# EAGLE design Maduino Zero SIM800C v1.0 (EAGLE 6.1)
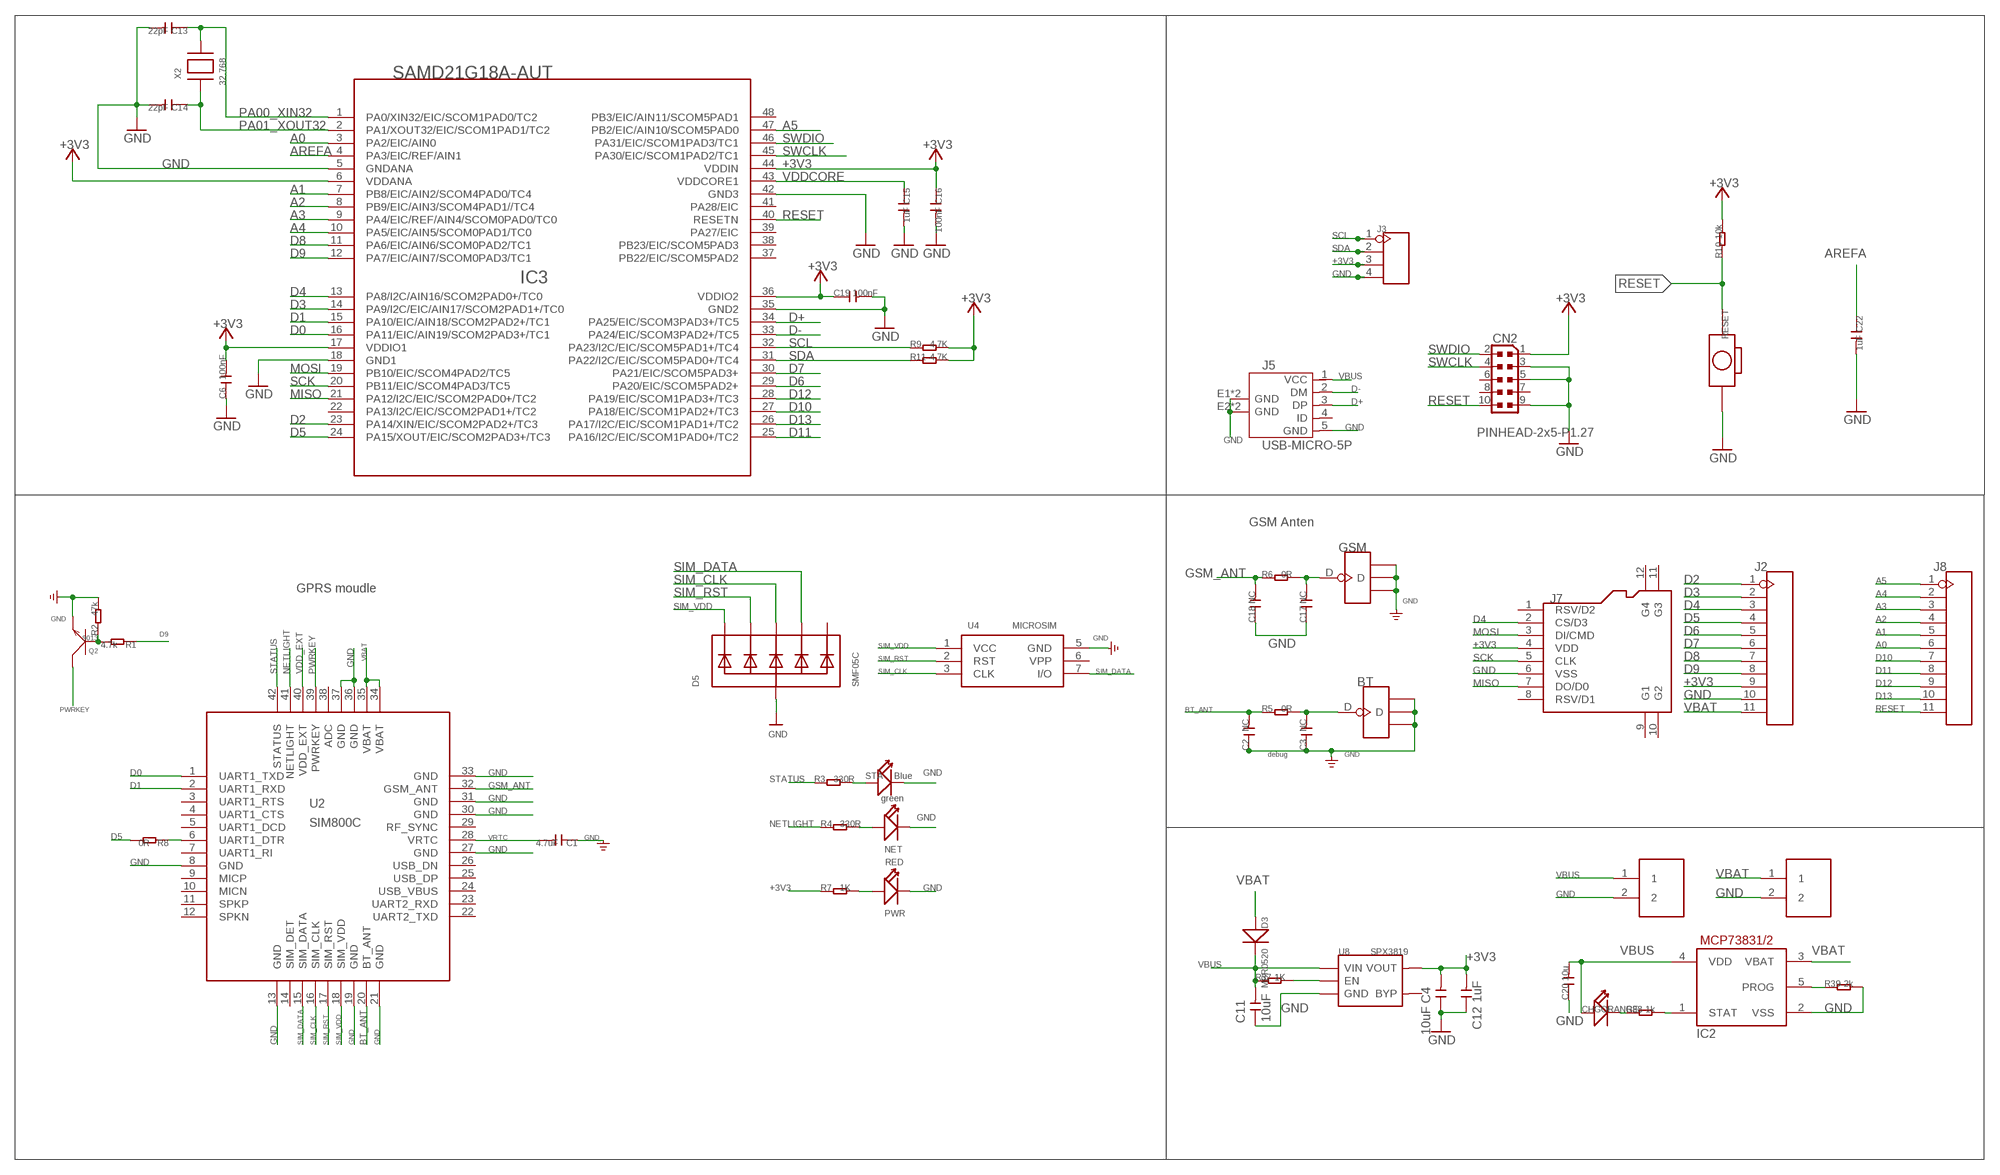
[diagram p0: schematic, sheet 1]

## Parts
BT  ANTENNA-U-FL  [4P-U-FL]
C1  4.7uF  C-0805  [C0805]
C2  NC  C-0402  [C0402]
C3  NC  C-0402  [C0402]
C4  10uF  C-0603  [C0603]
C6  100nF  C-0603  [C0603]
C11  10uF  C-0603  [C0603]
C12  1uF  C-0603  [C0603]
C13  22pF  C-0603  [C0603]
C14  22pF  C-0603  [C0603]
C15  1uF  C-0603  [C0603]
C16  100nF  C-0603  [C0603]
C17  NC  C-0402  [C0402]
C18  NC  C-0402  [C0402]
C19  100nF  C-0603  [C0603]
C20  10u  C-0603  [C0603]
C22  1uF  C-0603  [C0603]
CHG  ORANGE  007-LED0603  [D0603]
CN2  PINHEAD-2x5-P1.27  0171_PH127-205DF055G00AROUND-PADS  [PINHEAD_2X05_127]
D3  MBR0520  D'1206'  [SOD123]
D5  SMF05C  TVSARRAY_5LANE  [SOT363]
GSM  ANTENNA-U-FL  [4P-U-FL]
IC2  MCP73831/OT  [SOT23-5L]
IC3  SAMD21G18A-AUT  ATSAMD21G18A-AUT  [TQFP48-7X7]
J1  PH2.0-2P-90-DIP  [PH2.0-2P-90-DIP]
J2  HEADER-11P-2.54  [11P-2.54]
J3  HEADER-4P-60/35MILROUND  [4P-65/35ROUND]
J5  USB-MICRO-5P  [MICRO-USB-5P]
J6  PH2.0-2P-90-DIP  [PH2.0-2P-90-DIP]
J7  HOLDER-MICROSD-8P  [8P-SMD]
J8  HEADER-11P-2.54  [11P-2.54]
NET  green  LED'0603'  [LED-0603]
PWR  RED  LED'0603'  [LED-0603]
Q2  9013  TRANSISTOR-NPN-SOT23  [SOT23]
R1  4.7k  R-0603  [R0603]
R2  47k  R-0603  [R0603]
R3  330R  R-0603  [R0603]
R4  330R  R-0603  [R0603]
R5  0R  R-0603  [R0603]
R6  0R  R-0603  [R0603]
R7  1K  R-0603  [R0603]
R8  0R  R-0603  [R0603]
R9  4.7K  R-0603  [R0603]
R10  10k  R-0603  [R0603]
R11  4.7K  R-0603  [R0603]
R37  1K  R-0603  [R0603]
R38  1k  R-0603  [R0603]
R39  2k  R-0603  [R0603]
RESET  BOTTON-2P-90D  [2P-7.62X3.56-90D]
STA  Blue  LED'0603'  [LED-0603]
U2  SIM800C  [SIM800C]
U4  MICROSIM  [MICROSIM]
U8  SPX3819  [SOT23-5]
X2  32.768  XTAL-3.2X1.5  [XTAL3215]

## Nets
+3V3: C4.2 C6.2 C12.2 C16.1 C19.1 CN2.1 IC3.6(VDDANA) IC3.17(VDDIO1) IC3.36(VDDIO2) IC3.44(VDDIN) J2.9 J3.3 J7.4(VDD) R7.1 R9.2 R10.2 R11.2 U8.5(VOUT)
A0: IC3.3(PA2/EIC/AIN0) J8.6
A1: IC3.7(PB8/EIC/AIN2/SCOM4PAD0/TC4) J8.5
A2: IC3.8(PB9/EIC/AIN3/SCOM4PAD1//TC4) J8.4
A3: IC3.9(PA4/EIC/REF/AIN4/SCOM0PAD0/TC0) J8.3
A4: IC3.10(PA5/EIC/AIN5/SCOM0PAD1/TC0) J8.2
A5: IC3.47(PB2/EIC/AIN10/SCOM5PAD0) J8.1
AREFA: C22.1 IC3.4(PA3/EIC/REF/AIN1)
BT_ANT: C2.2 R5.1 U2.20(BT_ANT)
D0: IC3.16(PA11/EIC/AIN19/SCOM2PAD3+/TC1) U2.1(UART1_TXD)
D1: IC3.15(PA10/EIC/AIN18/SCOM2PAD2+/TC1) U2.2(UART1_RXD)
D2: IC3.23(PA14/XIN/EIC/SCOM2PAD2+/TC3) J2.1
D3: IC3.14(PA9/I2C/EIC/AIN17/SCOM2PAD1+/TC0) J2.2
D4: IC3.13(PA8/I2C/AIN16/SCOM2PAD0+/TC0) J2.3 J7.2(CS/D3)
D5: IC3.24(PA15/XOUT/EIC/SCOM2PAD3+/TC3) J2.4 R8.2
D6: IC3.29(PA20/EIC/SCOM5PAD2+) J2.5
D7: IC3.30(PA21/EIC/SCOM5PAD3+) J2.6
D8: IC3.11(PA6/EIC/AIN6/SCOM0PAD2/TC1) J2.7
D9: IC3.12(PA7/EIC/AIN7/SCOM0PAD3/TC1) J2.8 R1.1
D10: IC3.27(PA18/EIC/SCOM1PAD2+/TC3) J8.7
D11: IC3.25(PA16/I2C/EIC/SCOM1PAD0+/TC2) J8.8
D12: IC3.28(PA19/EIC/SCOM1PAD3+/TC3) J8.9
D13: IC3.26(PA17/I2C/EIC/SCOM1PAD1+/TC2) J8.10
D+: IC3.34(PA25/EIC/SCOM3PAD3+/TC5) J5.3(DP)
D-: IC3.33(PA24/EIC/SCOM3PAD2+/TC5) J5.2(DM)
GND: BT.GND1 BT.GND2 BT.GND3 C1.1 C2.1 C3.1 C4.1 C6.1 C11.1 C12.1 C13.2 C14.2 C15.2 C16.2 C17.1 C18.1 C19.2 C20.1 C22.2 CN2.3 CN2.5 CN2.9 D5.2(A) GSM.GND1 GSM.GND2 GSM.GND3 IC2.2(VSS) IC3.5(GNDANA) IC3.18(GND1) IC3.35(GND2) IC3.42(GND3) J1.2 J2.10 J3.4 J5.5(GND) J5.E1(GND) J5.E2(GND) J5.P1(GND) J5.P2(GND) J6.2 J7.6(VSS) NET.- PWR.- Q2.2(E) R2.2 R39.2 RESET.P$2 STA.- U2.8(GND) U2.13(GND) U2.19(GND) U2.21(GND) U2.27(GND) U2.30(GND) U2.31(GND) U2.33(GND) U2.36(GND) U2.37(GND) U4.5(GND) U8.2(GND)
GSM_ANT: C18.2 R6.1 U2.32(GSM_ANT)
MISO: IC3.21(PA12/I2C/EIC/SCOM2PAD0+/TC2) J7.7(DO/D0)
MOSI: IC3.19(PB10/EIC/SCOM4PAD2/TC5) J7.3(DI/CMD)
N$1: NET.+ R4.2
N$2: R8.1 U2.6(UART1_DTR)
N$3: PWR.+ R7.2
N$7: R3.2 STA.+
N$24: R37.2 U8.3(EN)
N$25: CHG.- R38.1
N$26: IC2.1(STAT) R38.2
N$28: BT.D C3.2 R5.2
N$31: IC2.5(PROG) R39.1
N$36: Q2.1(B) R1.2 R2.1
N$94: C17.2 GSM.D R6.2
NETLIGHT: R4.1 U2.41(NETLIGHT)
PA00_XIN32: C13.1 IC3.1(PA0/XIN32/EIC/SCOM1PAD0/TC2) X2.P$2
PA01_XOUT32: C14.1 IC3.2(PA1/XOUT32/EIC/SCOM1PAD1/TC2) X2.P$1
PWRKEY: Q2.3(C) U2.39(PWRKEY)
RESET: CN2.10 IC3.40(RESETN) J8.11 R10.1 RESET.P$1
SCK: IC3.20(PB11/EIC/SCOM4PAD3/TC5) J7.5(CLK)
SCL: IC3.32(PA23/I2C/EIC/SCOM5PAD1+/TC4) J3.1 R9.1
SDA: IC3.31(PA22/I2C/EIC/SCOM5PAD0+/TC4) J3.2 R11.1
SIM_CLK: D5.4(C3) U2.16(SIM_CLK) U4.3(CLK)
SIM_DATA: D5.5(C4) U2.15(SIM_DATA) U4.7(I/O)
SIM_RST: D5.3(C2) U2.17(SIM_RST) U4.2(RST)
SIM_VDD: D5.1(C1) U2.18(SIM_VDD) U4.1(VCC)
STATUS: R3.1 U2.42(STATUS)
SWCLK: CN2.4 IC3.45(PA30/EIC/SCOM1PAD2/TC1)
SWDIO: CN2.2 IC3.46(PA31/EIC/SCOM1PAD3/TC1)
VBAT: D3.+ IC2.3(VBAT) J2.11 J6.1 U2.34(VBAT) U2.35(VBAT)
VBUS: C11.2 C20.2 CHG.+ D3.- IC2.4(VDD) J1.1 J5.1(VCC) R37.1 U8.1(VIN)
VDD_EXT: U2.40(VDD_EXT)
VDDCORE: C15.1 IC3.43(VDDCORE1)
VRTC: C1.2 U2.28(VRTC)
Unconnected: CN2.6 CN2.7 CN2.8 D5.6(C5) IC3.22(PA13/I2C/EIC/SCOM2PAD1+/TC2) IC3.37(PB22/EIC/SCOM5PAD2) IC3.38(PB23/EIC/SCOM5PAD3) IC3.39(PA27/EIC) IC3.41(PA28/EIC) IC3.48(PB3/EIC/AIN11/SCOM5PAD1) J5.4(ID) J7.1(RSV/D2) J7.8(RSV/D1) J7.9(G1) J7.10(G2) J7.11(G3) J7.12(G4) U2.3(UART1_RTS) U2.4(UART1_CTS) U2.5(UART1_DCD) U2.7(UART1_RI) U2.9(MICP) U2.10(MICN) U2.11(SPKP) U2.12(SPKN) U2.14(SIM_DET) U2.22(UART2_TXD) U2.23(UART2_RXD) U2.24(USB_VBUS) U2.25(USB_DP) U2.26(USB_DN) U2.29(RF_SYNC) U2.38(ADC) U4.6(VPP) U8.4(BYP)

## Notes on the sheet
- GSM Anten
- GPRS moudle
- debug

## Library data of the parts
BT GSM = Connector:ANTENNA-U-FL
C1-C4 C6 C11-C20 C22 = Discrete:C*: Ceramic Capacitors
CHG = Discrete:007-LED*
CN2 = Connettori:0171_PH127-205DF055G00A: 2x5 PASSO 1,27
D3 = Discrete:D*
D5 = microbuilder:TVSARRAY_5LANE: Voltage Transient Suppressor Array SOT363 SMF05C - 100W 5V: Digikey - SMF05CT1GOSCT-ND
IC2 = adafruit:MCP73831: MCP73831/2 Miniature Single-Cell, Fully Integrated Li-Ion, Li-Polymer Charge Management Controllers. Nice and small simple lipoly charge controller, with adjustable current and status output (LED) http://www.ladyada.net/library/pcb/eaglelibrary.html
IC3 = IC:ATSAMD21G18A-AUT: Atmel D21 32bit ARM Cortex-M0 microcontroller - 48 PIN TQFP 256KB flash memory + 32KB SRAM
J1 J6 = Connector:PH2.0-2P-90-DIP
J2 J8 = Connector:HEADER-11P
J3 = Connector:HEADER-4P
J5 = Connector:USB-MICRO-5P
J7 = Connector:HOLDER-MICROSD-8P
NET PWR STA = Discrete:LED*
Q2 = Discrete:TRANSISTOR-NPN*: NPN audion
R1-R11 R37-R39 = Discrete:R*
RESET = Discrete:BOTTON-2P
U2 = moudle:SIM800C
U4 = Connector:MICROSIM
U8 = IC:SPX3819
X2 = adafruit2:XTAL: Low cost SMT crystals, no capacitors included

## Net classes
0 default: width 0.152 mm, drill 0.152 mm, clearance 0.152 mm
2 gnd: width 0.305 mm, drill 0.559 mm, clearance 0.254 mm
3 usbvcc: width 0.508 mm, drill 0.61 mm, clearance 0.254 mm
4 USBpair: width 0.254 mm, drill 0.406 mm, clearance 0.406 mm

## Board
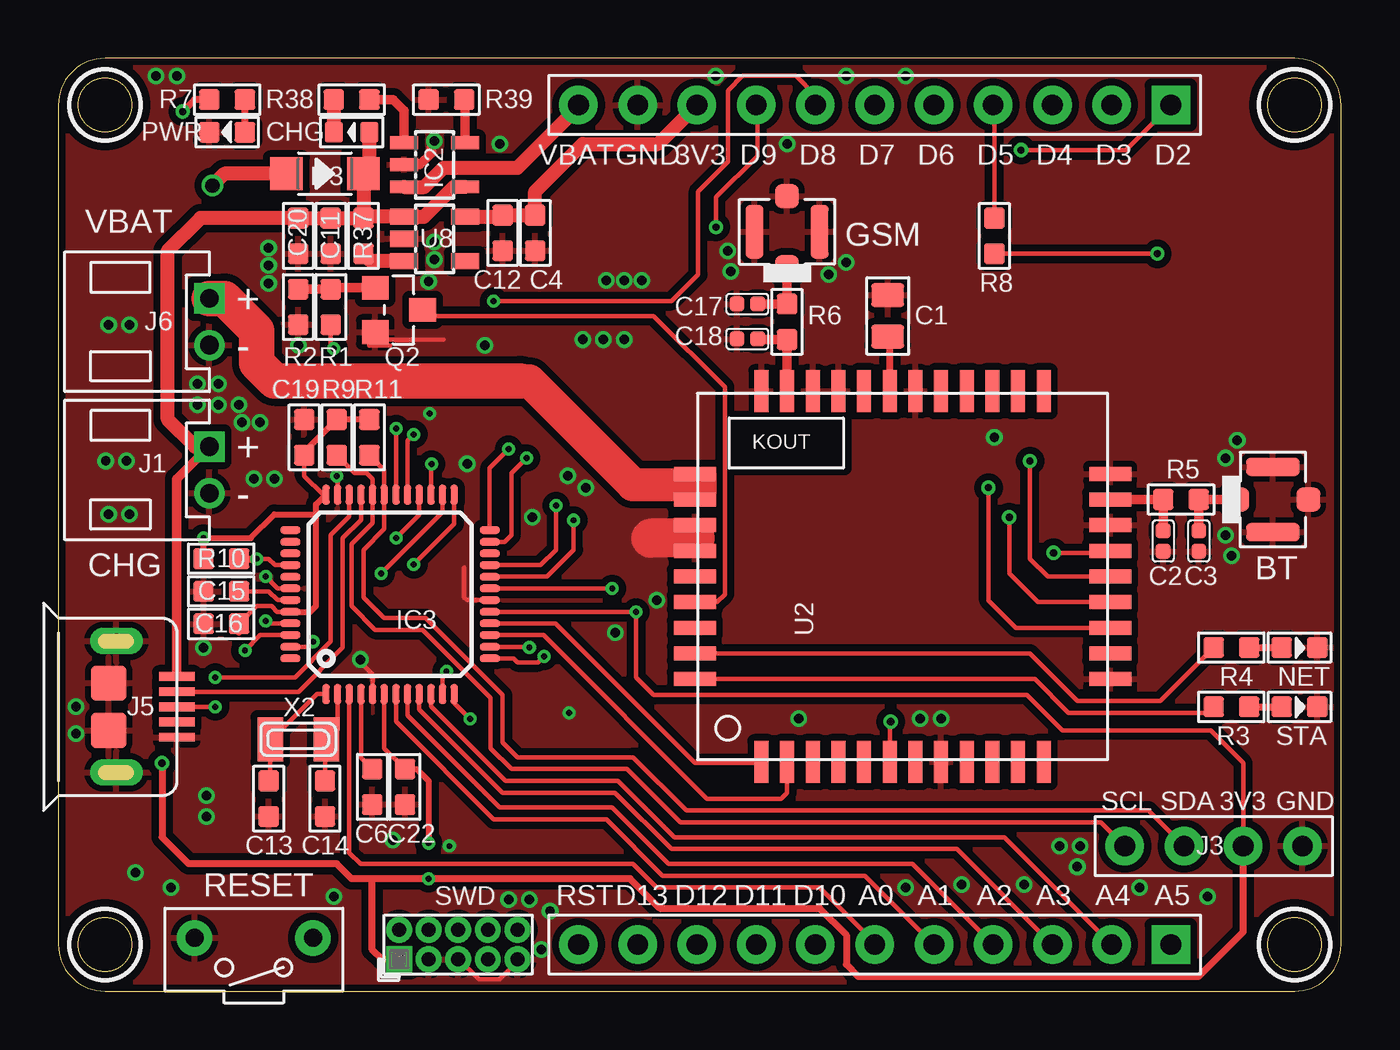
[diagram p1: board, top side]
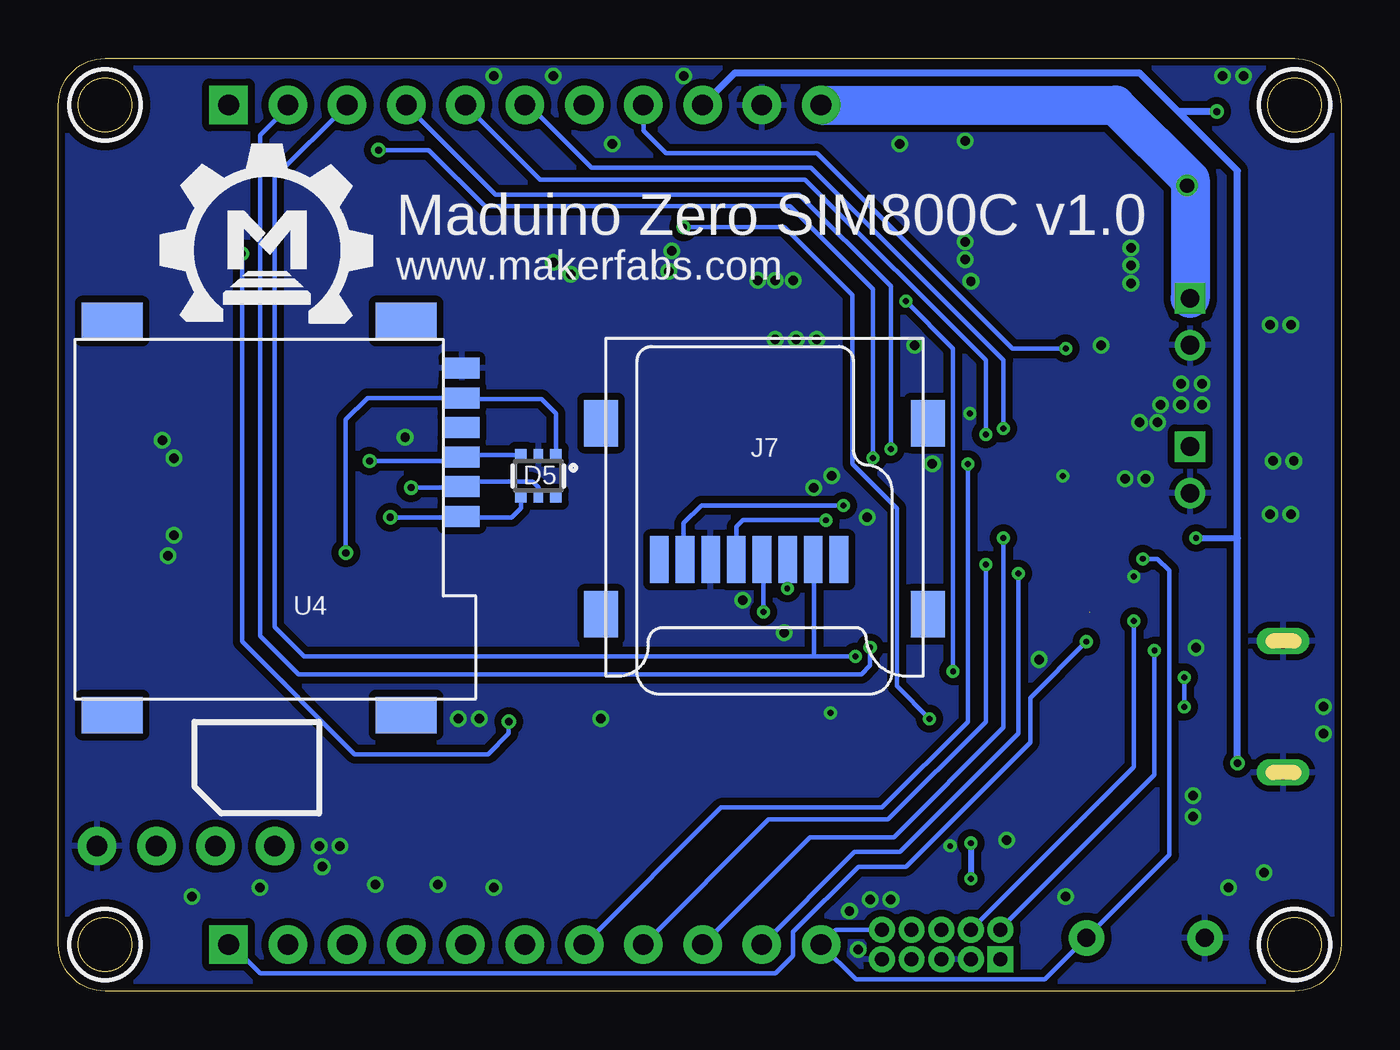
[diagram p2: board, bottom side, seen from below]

Size 55 x 40 mm. Coordinates in mm from the lower left corner, seen from the top.
Outline: 0,38 0,2 arc90 2,0 53,0 arc90 55,2 55,38 arc90 53,40 2,40 arc90 0,38
Outline: circle at 53,2 radius 1.14
Outline: circle at 53,38 radius 1.14
Outline: circle at 2,2 radius 1.14
Outline: circle at 2,38 radius 1.14
Copper layers (1*16): Top 0.035mm / dielectric 1.5mm / Bottom 0.035mm
Design rules: minimum track width 6mil, minimum drill 10mil, track to track 6mil, track to pad 6mil, pad to pad 6mil, via to via 6mil, smd to smd 0mil, copper to edge 10mil, drill to drill 10mil, minimum pad ring 10mil, minimum via ring 6mil, stop-mask expansion 2mil, vias tented up to drill 100mil, thermal gap 10mil
tRestrict: area 51.5,0.5 to 54.5,3.5; area 51.5,36.5 to 54.5,39.5; area 0.5,0.5 to 3.5,3.5; area 0.5,36.5 to 3.5,39.5
bRestrict: area 51.5,0.5 to 54.5,3.5; area 51.5,36.5 to 54.5,39.5; area 0.5,0.5 to 3.5,3.5; area 0.5,36.5 to 3.5,39.5

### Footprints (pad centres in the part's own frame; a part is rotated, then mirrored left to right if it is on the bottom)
4P-U-FL = smd 1.016 x 1.016: D -1.524,0; GND3 1.524,0 | smd 2.286 x 0.762: GND1 0,1.397; GND2 0,-1.397
C0805 = smd 1.016 x 1.397: 1 -0.889,0; 2 0.889,0
C0402 = smd 0.635 x 0.635: 1 -0.445,0; 2 0.445,0
C0603 = smd 0.889 x 0.889: 1 -0.762,0; 2 0.762,0
D0603 = smd 0.762 x 0.889: + -0.762,0; - 0.762,0
PINHEAD_2X05_127 = drill 0.6 pad 1.016 square: 1 -0.635,2.54 | drill 0.6 pad 1.016: 2 0.635,2.54; 3 -0.635,1.27; 4 0.635,1.27; 5 -0.635,0; 6 0.635,0; 7 -0.635,-1.27; 8 0.635,-1.27; 9 -0.635,-2.54; 10 0.635,-2.54
SOD123 = smd 1.397 x 1.397: + -1.651,0; - 1.651,0
SOT363 = smd 0.5 x 0.5: 1 -0.75,-0.9; 3 0.75,-0.9; 4 0.75,0.9; 6 -0.75,0.9 | smd 0.4 x 0.5: 2 0,-0.9; 5 0,0.9
SOT23-5L = smd 0.55 x 1.2: 1 -0.95,-1.3; 2 0,-1.3; 3 0.95,-1.3; 4 0.95,1.3; 5 -0.95,1.3
TQFP48-7X7 = smd 0.85 x 0.32: 1 -4.275,2.75; 2 -4.275,2.25; 3 -4.275,1.75; 4 -4.275,1.25; 5 -4.275,0.75; 6 -4.275,0.25; 7 -4.275,-0.25; 8 -4.275,-0.75; 9 -4.275,-1.25; 10 -4.275,-1.75; 11 -4.275,-2.25; 12 -4.275,-2.75; 25 4.275,-2.75; 26 4.275,-2.25; 27 4.275,-1.75; 28 4.275,-1.25; 29 4.275,-0.75; 30 4.275,-0.25; 31 4.275,0.25; 32 4.275,0.75; 33 4.275,1.25; 34 4.275,1.75; 35 4.275,2.25; 36 4.275,2.75 | smd 0.32 x 0.85: 13 -2.75,-4.275; 14 -2.25,-4.275; 15 -1.75,-4.275; 16 -1.25,-4.275; 17 -0.75,-4.275; 18 -0.25,-4.275; 19 0.25,-4.275; 20 0.75,-4.275; 21 1.25,-4.275; 22 1.75,-4.275; 23 2.25,-4.275; 24 2.75,-4.275; 37 2.75,4.275; 38 2.25,4.275; 39 1.75,4.275; 40 1.25,4.275; 41 0.75,4.275; 42 0.25,4.275; 43 -0.25,4.275; 44 -0.75,4.275; 45 -1.25,4.275; 46 -1.75,4.275; 47 -2.25,4.275; 48 -2.75,4.275
PH2.0-2P-90-DIP = drill 0.8 square: 1 0,1 | drill 0.8: 2 0,-1
11P-2.54 = drill 0.889 pad 1.651 square: 1 0,12.7 | drill 0.889 pad 1.651: 2 0,10.16; 3 0,7.62; 4 0,5.08; 5 0,2.54; 6 0,0; 7 0,-2.54; 8 0,-5.08; 9 0,-7.62; 10 0,-10.16; 11 0,-12.7
4P-65/35ROUND = drill 0.889 pad 1.651: 1 0,3.81; 2 0,1.27; 3 0,-1.27; 4 0,-3.81
MICRO-USB-5P = smd 0.38 x 1.52: 1 -1.3,0; 2 -0.65,0; 3 0,0; 4 0.65,0; 5 1.3,0 | smd 1.524 x 1.524: E1 -1.016,-2.921; E2 1.016,-2.921 | drill 0.635 pad 1.143 long: P1 -2.819,-2.591; P2 2.819,-2.591
8P-SMD = smd 0.8 x 2.008: 1 -3.198,0.254; 2 -2.098,0.254; 3 -0.998,0.254; 4 0.102,0.254; 5 1.202,0.254; 6 2.302,0.254; 7 3.402,0.254; 8 4.502,0.254 | smd 1.45 x 2: 9 -7.002,2.6; 10 7.002,2.6; 11 -7.002,-5.598; 12 7.002,-5.598
LED-0603 = smd 0.889 x 0.889: + -0.762,0; - 0.762,0
SOT23 = smd 1.016 x 1.143: 1 -0.95,-1.016; 2 0.95,-1.016; 3 0,1.016
R0603 = smd 0.889 x 0.889: 1 -0.762,0; 2 0.762,0
2P-7.62X3.56-90D = drill 0.762 pad 1.524: P$1 0,2.54; P$2 0,-2.54
SIM800C = smd 1.8 x 0.6: 1 -7.95,6.05; 2 -7.95,4.95; 3 -7.95,3.85; 4 -7.95,2.75; 5 -7.95,1.65; 6 -7.95,0.55; 7 -7.95,-0.55; 8 -7.95,-1.65; 9 -7.95,-2.75; 10 -7.95,-3.85; 11 -7.95,-4.95; 12 -7.95,-6.05; 22 7.95,-6.05; 23 7.95,-4.95; 24 7.95,-3.85; 25 7.95,-2.75; 26 7.95,-1.65; 27 7.95,-0.55; 28 7.95,0.55; 29 7.95,1.65; 30 7.95,2.75; 31 7.95,3.85; 32 7.95,4.95; 33 7.95,6.05 | smd 0.6 x 1.8: 13 -4.4,-8.9; 14 -3.3,-8.9; 15 -2.2,-8.9; 16 -1.1,-8.9; 17 0,-8.9; 18 1.1,-8.9; 19 2.2,-8.9; 20 3.3,-8.9; 21 4.4,-8.9; 34 4.4,8.9; 35 3.3,8.9; 36 2.2,8.9; 37 1.1,8.9; 38 0,8.9; 39 -1.1,8.9; 40 -2.2,8.9; 41 -3.3,8.9; 42 -4.4,8.9
MICROSIM = smd 1.5 x 0.9: 1 -0.8,2.5; 2 -0.8,5.04; 3 -0.8,7.58; 5 -0.8,1.23; 6 -0.8,3.77; 7 -0.8,6.31 | smd 2.61 x 1.56: P$1 1.6,-0.8; P$2 14.2,-0.8; P$3 14.2,16.1; P$4 1.6,16.1
SOT23-5 = smd 0.69 x 1.2: 1 -0.95,-1.3; 2 0,-1.3; 3 0.95,-1.3; 4 0.95,1.3; 5 -0.95,1.3
XTAL3215 = smd 1.1 x 1.9: P$1 1.2,0; P$2 -1.2,0

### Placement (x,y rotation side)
BT  52.07,21.08 0 top
C1  35.56,28.96 270 top
C2  47.37,19.3 90 top
C3  48.9,19.3 90 top
C4  20.45,32.51 90 top
C6  14.86,8.76 90 top
C11  11.68,32.38 90 top
C12  19.05,32.51 90 top
C13  9.02,8.26 270 top
C14  11.43,8.26 270 top
C15  6.99,17.14 180 top
C16  6.99,15.75 180 top
C17  29.54,29.46 0 top
C18  29.54,27.97 0 top
C19  10.54,23.75 90 top
C20  10.29,32.38 90 top
C22  13.46,8.76 270 top
CHG  12.57,36.83 180 top
CN2  17.14,2 90 top
D3  11.43,35.05 0 top
D5  34.42,22.1 180 bottom
GSM  31.24,32.56 90 top
IC2  16.13,35.43 270 top
IC3  14.22,17.02 90 top
J1  6.48,22.35 0 top
J2  35,38 270 top
J3  49.53,6.22 90 top
J5  5.08,12.19 270 top
J6  6.48,28.7 0 top
J7  24.73,18.76 180 bottom
J8  35,2 270 top
NET  53.21,14.73 0 top
PWR  7.24,36.83 180 top
Q2  14.61,29.21 270 top
R1  11.68,29.34 90 top
R2  10.29,29.34 270 top
R3  50.29,12.19 0 top
R4  50.29,14.73 0 top
R5  48.13,21.08 0 top
R6  31.24,28.7 90 top
R7  7.24,38.23 0 top
R8  40.13,32.38 90 top
R9  11.94,23.75 90 top
R10  6.99,18.54 180 top
R11  13.34,23.75 90 top
R37  13.08,32.38 270 top
R38  12.57,38.23 0 top
R39  16.64,38.23 180 top
RESET  8.38,2.29 270 top
STA  53.21,12.19 0 top
U2  36.2,17.78 90 top
U4  38.49,27.94 180 bottom
U8  16.13,32.26 270 top
U$1  [MAKERFABS_0.3]  50.17,28.7 0 bottom
X2  10.29,10.79 0 top

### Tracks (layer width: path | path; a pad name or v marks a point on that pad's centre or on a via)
+3V3  (via drill 0.25, 0.3)  (1 unrouted)
  Top 0.203: IC3.6 13.97,10.41 C6.2 | IC3.36 11.35,21.29 10.54,22.1 C19.1 | IC3.44 9.39,16.27 9.14,16.51 8.51,16.51 C16.1 | IC3.17 24.75,16.27 v24.77,16.26 24.77,13.46 25.53,12.7 41.53,12.7 43.05,11.18 49.4,11.18 50.8,9.78 J3.3
  Top 0.254: 10.81,16.27 11.05,16.51 11.05,20.45 | 11.05,20.45 11.05,20.87 IC3.36 | R11.2 R9.2 10.54,23.11 C19.1 | C16.1 7.75,15.37 | IC3.44 10.78,16.27 10.79,16.26 | v15.88,6.35 15.88,9.02 15.37,9.53 C6.2 | R10.2 v6.22,19.43 8.26,19.43 9.27,20.45 11.05,20.45
  Top 0.305: v4.45,9.78 4.45,6.6 5.59,5.46 11.94,5.46 12.57,4.83 13.46,4.83 | CN2.1 13.88,1.36 13.46,1.78 13.46,4.83 | 13.46,4.83 v15.88,4.83 24.51,4.83 25.78,3.56 32.64,3.56 33.78,2.41 33.78,1.14 34.29,0.64 48.9,0.64 50.8,2.54 J3.3 | R7.1 5.84,38.23 v5.33,37.72
  Top 0.61: J2.9 25.7,36.32 22.48,36.32 20.45,34.29 C4.2 C12.2 18.98,33.21 U8.5
  Bottom 0.203: v24.77,16.26 24.77,18.54 24.87,18.54 | 24.89,18.54 24.87,18.54 | 24.87,18.54 J7.4
  Bottom 0.254: 24.89,18.44 J7.4 | v15.88,6.35 v15.88,4.83 | v6.22,19.43 4.45,19.43
  Bottom 0.305: v4.45,9.78 4.45,19.43 4.45,35.18 6.99,37.72 | 6.99,37.72 8.64,39.37 26.01,39.37 J2.9 | v5.33,37.72 6.99,37.72
A0
  Top 0.203: J8.6 35.02,2 35.05,2.03 32.64,4.45 25.65,4.45 24.64,5.46 12.95,5.46 12.47,5.94 IC3.3
A1
  Top 0.203: IC3.7 14.47,11.56 18.67,7.37 23.5,7.37 25.91,4.95 34.59,4.95 J8.5
A2
  Top 0.203: IC3.8 14.97,11.82 18.92,7.87 23.75,7.87 26.16,5.46 36.62,5.46 J8.4
A3
  Top 0.203: IC3.9 15.47,12.09 19.05,8.51 23.88,8.51 26.29,6.1 38.52,6.1 J8.3
A4
  Top 0.203: IC3.10 15.97,12.22 19.18,9.02 24,9.02 26.42,6.6 40.56,6.6 J8.2
A5  (via drill 0.25)
  Top 0.203: IC3.47 10.7,14.77 v10.92,14.99
  Bottom 0.203: J8.1 47.59,2 46.35,0.76 24.26,0.76 23.5,1.52 23.5,2.54 20.7,5.33 18.67,5.33 13.34,10.67 13.34,12.57 v10.92,14.99
AREFA
  Top 0.203: IC3.4 12.97,10.01 C22.1
BT_ANT
  Top 0.406: U2.20 R5.1 C2.2
D0
  Top 0.203: IC3.16 21.32,15.77 27.3,9.78 30.09,9.78 U2.1
D1
  Top 0.203: IC3.15 20.8,15.27 27.81,8.26 30.99,8.26 31.24,8.51 U2.2
D2  (via drill 0.25, 0.3)
  Top 0.203: IC3.23 19.14,19.27 19.43,19.56 19.43,22.23 v20.07,22.86 | v41.27,36.07 45.77,36.07 J2.1
  Bottom 0.203: v20.07,22.86 20.07,30.1 23.62,33.66 36.7,33.66 39.12,36.07 v41.27,36.07
D3  (via drill 0.25)
  Top 0.203: IC3.14 20.16,14.77 v20.19,14.73
  Bottom 0.203: v20.19,14.73 20.19,13.97 20.57,13.59 44.7,13.59 46.35,15.24 46.35,36.7 45.09,37.97 45.16,37.97 J2.2
D4  (via drill 0.25)
  Top 0.203: IC3.13 19.51,14.27 19.68,14.1 20.57,14.1 v20.83,14.35
  Bottom 0.203: v20.83,14.35 22.61,14.35 | 22.61,14.35 44.45,14.35 45.72,15.62 45.72,34.9 J2.3 | J7.2 22.63,18.52 22.61,18.54 22.61,14.35
D5  (via drill 0.25)
  Top 0.203: IC3.24 18.5,22.44 v19.3,23.24 | R8.2 40.13,37.97 40.11,37.97 J2.4
  Bottom 0.203: v19.3,23.24 19.3,30.23 23.24,34.16 36.24,34.16 J2.4
D6  (via drill 0.25)
  Top 0.203: IC3.29 14.97,23.61 v15.24,23.88
  Bottom 0.203: v15.24,23.88 15.24,27.05 22.99,34.8 34.34,34.8 J2.5
D7  (via drill 0.25)
  Top 0.203: IC3.30 v14.47,24.13 v14.48,24.13
  Bottom 0.203: v14.48,24.13 14.48,27.05 22.73,35.31 32.13,35.31 34.92,38.1 34.92,37.97
  Bottom 0.254: 34.92,37.97 34.97,37.97 J2.6
D8  (via drill 0.25)
  Top 0.203: IC3.11 16.47,13.55 v16.64,13.72 | J2.7 32.46,38.41 31.62,39.24 29.34,39.24 28.7,38.61 28.7,35.56 27.43,34.29 27.43,30.73 26.29,29.59 v18.67,29.59
  Bottom 0.203: v16.64,13.72 16.64,27.56 v18.67,29.59
D9  (via drill 0.25, 0.3)
  Top 0.203: IC3.12 16.97,12.36 v17.65,11.68 | v28.19,32.77 28.19,34.04 29.97,35.81 29.97,37.95 J2.8 | R1.1 11.68,27.69 v11.81,27.56
  Bottom 0.203: J2.8 29.92,36.91 28.96,35.94 22.48,35.94 14.1,27.56 v11.81,27.56 | v17.65,11.68 19.05,13.08 19.05,20.7 20.95,22.61 20.95,29.84 23.88,32.77 v28.19,32.77
D10  (via drill 0.25)
  Top 0.203: IC3.27 15.97,22.58 v16,22.61
  Bottom 0.203: v16,22.61 16,11.56 19.68,7.87 26.59,7.87 J8.7
D11  (via drill 0.25)
  Top 0.203: IC3.25 16.97,20.02 v15.24,18.29
  Bottom 0.203: v15.24,18.29 15.24,11.56 19.43,7.37 24.55,7.37 J8.8
D12  (via drill 0.25)
  Top 0.203: IC3.28 15.47,20.43 v14.48,19.43
  Bottom 0.203: v14.48,19.43 14.48,11.3 19.18,6.6 22.78,6.6 J8.9
D13  (via drill 0.25)
  Top 0.203: IC3.26 16.47,20.54 v13.84,17.91
  Bottom 0.203: v13.84,17.91 13.84,11.05 18.92,5.97 20.87,5.97 J8.10
D+  (via drill 0.25)
  Top 0.203: IC3.34 12.47,20.35 11.68,19.56 11.68,14.99 10.16,13.46 v6.73,13.46 | v6.73,12.19 J5.3
  Bottom 0.203: v6.73,13.46 v6.73,12.19
D-
  Top 0.203: IC3.33 12.97,20.21 12.19,19.43 12.19,14.73 10.3,12.84 J5.2
GND  (via drill 0.25, 0.41)
  Top 0.203: IC3.35 11.97,22.06 v11.94,22.1 | IC3.5 13.47,13.58 12.83,14.22 | IC3.18 17.52,16.77 17.4,16.89 17.4,18.16 | 19.75,1.33 19.81,1.4 | CN2.9 19.72,1.36 19.75,1.33 | IC3.42 9.4,17.27 v8.89,17.78 | 16.51,27.94 13.72,27.94 13.72,27.81 13.59,27.69 | 14.22,27.69 13.59,27.69 | 13.59,27.69 13.34,27.69 | 19.75,1.33 18.92,0.51 18.03,0.51 17.14,1.4
  Top 0.406: IC2.2 15.49,35.43 16,35.94 16,36.32 v16.13,36.45
  Top 1.676: 27.3,19.43 25.4,19.43
  Bottom 0.203: v8.89,17.78 8.89,17.65 8.76,17.78
  other vias: 10.29,27.69 9.02,31.88 9.02,31.11 7.75,25.15 6.86,25.15 0.76,11.05 0.76,12.19 18.29,27.69 18.92,36.32 8.64,24.38 7.87,24.38 3.05,28.57 2.16,28.57 6.86,26.04 5.97,26.04 5.97,25.15 15.88,30.43 16.13,32.13 16.13,31.37 9.02,30.35 3.05,20.45 2.16,20.45 5.08,39.24 4.19,39.24 2.92,22.73 2.03,22.73 12.95,14.22 17.53,22.61 14.35,6.48 6.22,14.73 20.7,1.78 21.08,3.43 3.3,5.08 4.83,4.45 6.35,8.38 6.35,7.49 16.76,6.22 42.93,6.22 43.81,6.22 43.69,5.33 41.4,4.57 38.73,4.57 36.32,4.45 46.35,4.45 20.19,3.94 19.3,3.94 49.28,4.06 9.27,21.97 8.38,21.97 28.19,39.24 31.24,36.32 33.78,39.24 36.32,39.24 15.93,24.77 21.84,22.1 23.5,30.48 25.65,16.76 23.88,15.37 22.61,21.59 20.32,20.32 21.89,11.94 24.26,30.48 25.02,30.48 28.7,31.75 28.83,30.86 33.02,30.73 33.78,31.24 50.04,22.86 50.04,19.56 50.29,18.67 50.55,23.62 11.81,4.06 22.48,27.94 23.37,27.94 24.26,27.94 36.96,11.68 37.85,11.68 40.13,23.75 31.75,11.68
  pour Bottom (isolate 0.305): -1.27,-1.27 60,-1.27 60,45 -1.27,45
  pour Top (isolate 0.305): -1.27,-1.27 60,-1.27 60,45 -1.27,45
GSM_ANT
  Top 0.406: U2.32 R6.1 30.01,27.94 C18.2
MISO  (via drill 0.25)
  Top 0.203: IC3.21 20.68,18.27 21.34,18.92 v21.34,20.83
  Bottom 0.203: v21.34,20.83 27.43,20.83 28.19,20.07 28.19,18.41 28.13,18.48 J7.7
MOSI  (via drill 0.25)
  Top 0.203: IC3.19 v23.75,17.27
  Bottom 0.203: v23.75,17.27 23.75,18.48 J7.3
N$1
  Top 0.305: R4.2 NET.+
N$2  (via drill 0.3)
  Top 0.203: R8.1 v47.12,31.62 | U2.6 35.65,11.52 v35.69,11.56
  Bottom 0.203: v47.12,31.62 47.12,14.99 42.29,10.16 36.58,10.16 35.69,11.05 v35.69,11.56
N$3
  Top 0.305: PWR.+ R7.2
N$7
  Top 0.305: R3.2 STA.+
N$24
  Top 0.61: U8.3 13.4,31.31 R37.2
N$25
  Top 0.61: R38.1 CHG.-
N$26
  Top 0.406: IC2.1 14.83,37.75 14.35,38.23 R38.2
N$28
  Top 0.406: C3.2 R5.2 BT.D
N$31
  Top 0.406: IC2.5 17.43,38.2 R39.1
N$36
  Top 0.406: R2.1 R1.2 | Q2.1 11.74,30.16
  Top 0.61: 11.74,30.16 R1.2
N$94
  Top 0.406: GSM.D R6.2 C17.2
NETLIGHT
  Top 0.203: U2.41 41.65,14.48 43.69,12.45 47.24,12.45 R4.1
PA00_XIN32
  Top 0.203: IC3.1 11.09,12.74 9.14,10.79 X2.P$2 9.09,9.09 C13.1
PA01_XOUT32
  Top 0.203: IC3.2 11.97,11.21 11.49,10.72 | X2.P$1 11.49,10.72 | 11.49,10.72 11.43,10.67 C14.1
PWRKEY
  Top 0.203: U2.39 28.24,16.68 28.57,17.02 28.57,25.91 25.53,28.96 15.88,28.96 Q2.3
RESET  (via drill 0.25)
  Top 0.203: IC3.40 9.29,18.27 9.02,18.54 v8.51,18.54
  Top 0.305: R10.1 v8.51,18.54
  Bottom 0.203: CN2.10 21.66,2.63 J8.11 20.81,0.51 12.7,0.51 RESET.P$1 7.37,5.84 7.37,18.03 7.87,18.54 v8.51,18.54
SCK  (via drill 0.25)
  Top 0.203: IC3.20 20.95,17.78 22.1,18.92 v22.1,20.19
  Bottom 0.203: J7.5 25.93,19.92 25.65,20.19 v22.1,20.19
SCL
  Top 0.203: R9.1 12.7,22.23 13.21,22.23 13.47,21.96 IC3.32 13.47,20.08 12.57,19.18 12.57,16.51 13.59,15.49 15.62,15.49 18.54,12.57 18.54,10.41 19.43,9.53 24.38,9.53 26.67,7.24 44.7,7.24 J3.1
SDA
  Top 0.203: R11.1 13.97,22.35 IC3.31 13.97,19.82 13.08,18.92 13.08,16.89 13.97,16 15.75,16 19.05,12.7 19.05,10.67 19.68,10.03 24.64,10.03 26.92,7.75 46.74,7.75 J3.2
SIM_CLK  (via drill 0.3)
  Top 0.203: U2.16 41.99,16.68 40.77,17.91 v40.77,20.32
  Bottom 0.203: D5.4 35.17,20.71 35.56,20.32 37.65,20.32 U4.3 37.73,20.32 v40.77,20.32
  Bottom 0.305: 37.73,20.32 37.72,20.32
SIM_DATA  (via drill 0.3)
  Top 0.203: U2.15 41.06,15.58 39.88,16.76 v39.88,21.59
  Bottom 0.203: D5.5 34.42,21.59 34.67,21.84 37.48,21.84 U4.7 37.73,21.59 v39.88,21.59
SIM_RST  (via drill 0.3)
  Top 0.203: U2.17 42.42,17.78 41.66,18.54 v41.66,22.73
  Bottom 0.203: D5.3 37.59,23 U4.2 37.86,22.73 v41.66,22.73
SIM_VDD  (via drill 0.3)
  Top 0.203: v42.67,18.8 45.01,18.8 U2.18
  Bottom 0.203: D5.1 33.67,24.78 34.29,25.4 37.65,25.4 U4.1 41.74,25.44 42.67,24.51 v42.67,18.8
STATUS
  Top 0.203: U2.42 41.87,13.38 43.31,11.94 49.28,11.94 R3.1
SWCLK  (via drill 0.25)
  Top 0.203: IC3.45 9,15.77 v8.89,15.88
  Bottom 0.203: v8.89,15.88 8.89,9.62 CN2.4
SWDIO  (via drill 0.25)
  Top 0.203: IC3.46 8.66,15.27 v8,14.61
  Bottom 0.203: v8,14.61 8,9.27 14.61,2.67 CN2.2
VBAT  (via drill 0.61)
  Top 0.305: U2.34 27.86,22.18 27.94,22.1 28.07,22.23 28.07,21.34 27.94,21.21 27.81,21.21 27.43,21.59 | U2.35 27.3,21.35 26.92,21.72
  Top 0.61: J2.11 22.33,37.97 22.35,37.97 19.68,35.31 16.51,35.31 15.69,34.48 IC2.3 | D3.+ 7.11,35.05 v6.6,34.54
  Top 1.422: 19.81,26.16 20.19,26.16 24.64,21.72 26.92,21.72 27.3,21.72 27.43,21.59
  Top 1.524: J6.1 7.13,29.7 8.51,28.32 8.51,26.92 9.27,26.16 19.81,26.16
  Bottom 0.61: v6.6,34.54 6.48,34.54
  Bottom 1.676: J2.11 9.68,38 6.48,34.8 6.48,34.54 J6.1
VBUS
  Top 0.406: J5.1 5.08,21.95 J1.1
  Top 0.61: CHG.+ 13.34,34.8 D3.- R37.1 | J1.1 5.86,23.35 4.7,24.51 4.7,31.75 6.1,33.15 C20.2 C11.2 R37.1 | IC2.4 16.96,34.48 15.68,33.21 U8.1 13.14,33.21 R37.1
VDDCORE
  Top 0.203: IC3.43 9.39,16.77 9.02,17.14 C15.1
VRTC
  Top 0.305: U2.28 35.65,27.98 C1.2

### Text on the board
tPlace: VBAT | GND | 3V3 | D9 | D8 | D7 | D6 | D5 | D4 | D3 | D2 | VBAT | + | - | + | - | CHG | SCL | SDA | 3V3 | GND | SWD | RST | D13 | D12 | D11 | D10 | A0 | A1 | A2 | A3 | A4 | A5
bNames: Maduino Zero SIM800C v1.0 | www.makerfabs.com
